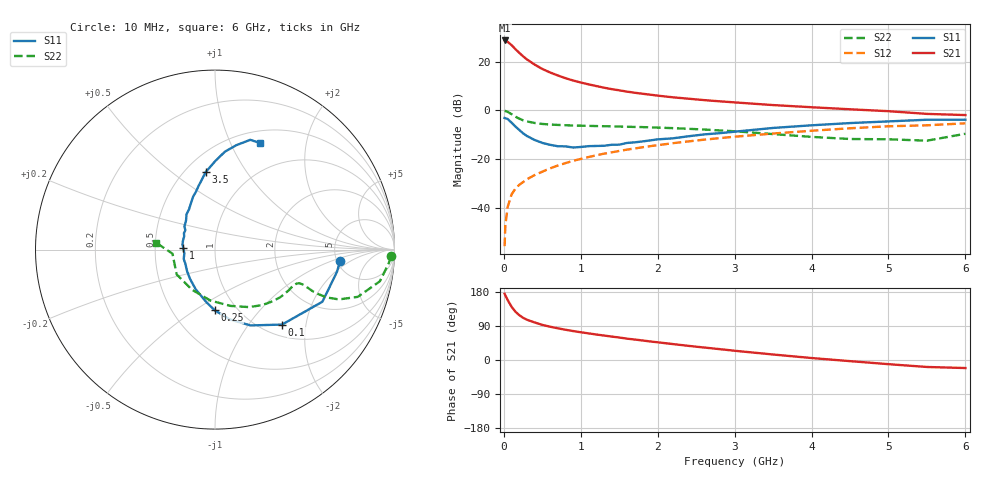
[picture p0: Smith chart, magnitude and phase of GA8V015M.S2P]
! Infineon Technologies  Discrete & RF Semiconductors
! BF775
! Si NPN RF Bipolar Junction Transistor in SOT23
! VCE = 8 V  IC = 15 mA
! Common Emitter S-Parameters:  May  1996
# GHz  S  MA  R  50
!  f  S11  S21  S12  S22
! GHz  MAG  ANG  MAG  ANG  MAG  ANG  MAG  ANG
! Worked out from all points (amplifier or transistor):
!   36 points, 10 MHz to 6 GHz, reference 50 ohm
!   highest |S21| = 28.8 dB at 10 MHz (marker M1)
!   |S21| within 3 dB of that: start of sweep to 133.2 MHz
!   unconditionally stable (mu >= 1): 498.7 MHz to 2.793 GHz
!   at 250 MHz: K = 0.76, MSG = 25.9 dB, |S12| = -29.5 dB
!   at 1.4 GHz: K = 1.09, MAG = 11.2 dB, |S12| = -17.3 dB
!   at 6 GHz: K = 0.90, MSG = 1.7 dB, |S12| = -5.3 dB
!   S11 on the Smith chart (normalised r, x): 10 MHz: 5.32, -1.35; 100 MHz: 1.21, -1.47; 250 MHz: 0.79, -0.60; 1 GHz: 0.70, +0.01; 3.5 GHz: 0.63, +0.67; 6 GHz: 0.64, +1.30
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0.01  0.7001 -5.3  27.59 174.8  0.0016 82.0  0.9823 -2.1
0.02  0.6906 -10.4  27.05 170.4  0.0044 83.7  0.9705 -4.6
0.05  0.6651 -25.9  25.78 158.1  0.0103 77.4  0.9352 -10.9
0.1  0.5603 -48.2  22.18 140.6  0.0186 71.0  0.8382 -18.3
0.15  0.4666 -64.9  18.32 127.5  0.0244 66.5  0.744 -21.9
0.2  0.3965 -78.3  15.37 118.5  0.0293 65.3  0.6765 -23.2
0.25  0.3377 -90.3  13.03 111.4  0.0334 65.0  0.6266 -23.3
0.3  0.2974 -99.2  11.24 106.3  0.0381 66.0  0.593 -23.1
0.4  0.2465 -115.7  8.788 99.1  0.0466 66.7  0.5522 -22.2
0.5  0.2143 -130.6  7.142 92.7  0.0547 67.8  0.5267 -21.7
0.6  0.1958 -142.9  6.057 87.9  0.0639 68.2  0.5124 -21.7
0.7  0.183 -154.2  5.254 83.7  0.0731 68.7  0.5028 -21.9
0.8  0.1819 -163.4  4.614 79.9  0.082 68.5  0.4951 -22.4
1  0.1766 177.6  3.754 73.2  0.1001 68.2  0.4848 -24.0
1.1  0.1837 170.8  3.444 70.3  0.1095 68.0  0.4809 -25.2
1.3  0.1868 156.8  2.944 64.6  0.1283 66.7  0.4724 -27.4
1.6  0.2135 143.0  2.439 56.4  0.1557 64.6  0.4607 -31.6
2.2  0.2664 123.0  1.861 42.0  0.2115 59.3  0.4315 -41.7
3.5  0.4354 96.8  1.288 14.5  0.3338 45.0  0.3254 -74.6
4.5  0.5486 84.2  1.055 -3.0  0.4286 32.7  0.2577 -120.0
5.5  0.6425 72.2  0.848 -18.4  0.4936 17.5  0.2379 -174.5
6  0.6443 67.0  0.802 -21.2  0.5425 13.3  0.3305 173.3
